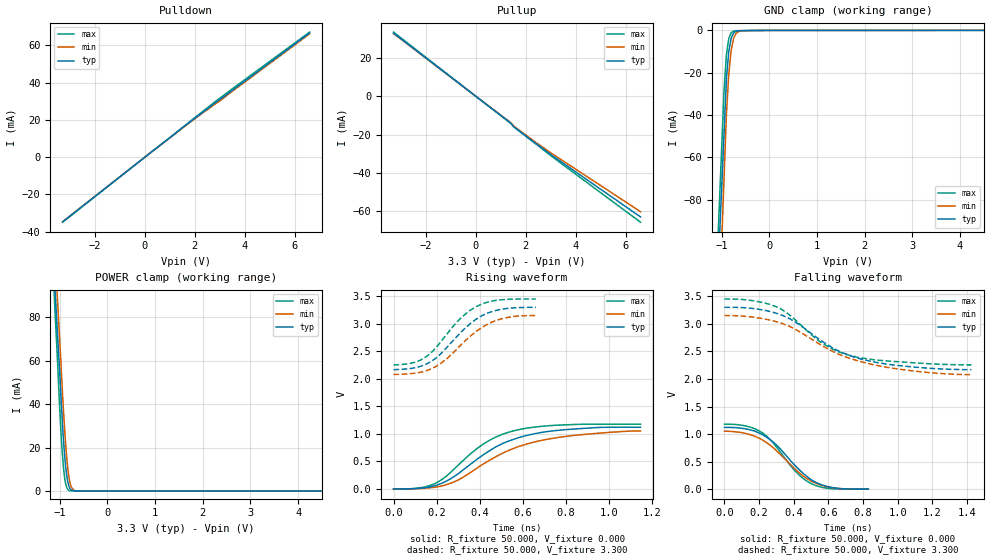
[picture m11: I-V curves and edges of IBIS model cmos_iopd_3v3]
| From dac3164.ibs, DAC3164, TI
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[Model]   cmos_iopd_3v3
Model_type I/O
Vinl=8.250E-01
Vinh=1.980E+00
Vref=0.000E+00
Rref=1.000E+06
Cref=0.000E+00
Vmeas=1.650E+00
C_comp   1.070E-12   1.070E-12   1.070E-12
[Voltage Range]   3.300E+00   3.150E+00   3.450E+00
[POWER Clamp Reference]   3.300E+00   3.150E+00   3.450E+00
[GND Clamp Reference]   0.000E+00   0.000E+00   0.000E+00
[Pullup Reference]   3.300E+00   3.150E+00   3.450E+00
[Pulldown Reference]   0.000E+00   0.000E+00   0.000E+00
[Temperature Range]   25   85   -40
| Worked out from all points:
|   slope of the pulldown table from 0 to 0.495 V, typ, clamps not added: 95.4 ohm
|   slope of the pullup table from 0 to 0.495 V, typ, clamps not added: 100 ohm
|   GND clamp passes 1 mA (typ) near -0.74 V on its own axis
|   POWER clamp passes 1 mA (typ) near -0.78 V on its own axis
|   rising waveform, R_fixture 50.000, V_fixture 0.000: 20-80 % time 273ps typ, 321ps min, 229ps max; typ from 0 V to 1.12 V
|   falling waveform, R_fixture 50.000, V_fixture 0.000: 20-80 % time 214ps typ, 223ps min, 189ps max; typ from 1.12 V to 0 V
|   rising waveform, R_fixture 50.000, V_fixture 3.300: 20-80 % time 178ps typ, 188ps min, 165ps max; typ from 2.17 V to 3.3 V
|   falling waveform, R_fixture 50.000, V_fixture 3.300: 20-80 % time 365ps typ, 424ps min, 305ps max; typ from 3.3 V to 2.17 V
[GND Clamp]
-3.3V     -1.265A    -1.499A    -1.32A
-950mV    -49.06mA   -70.33mA   -28.61mA
-900mV    -23.2mA    -39.94mA   -11.61mA
-850mV    -9.95mA    -20.84mA   -3.839mA
-800mV    -3.735mA   -9.456mA   -1.133mA
-750mV    -1.255mA   -3.879mA   -337.2uA
-700mV    -399.4uA   -1.494mA   -148.9uA
-650mV    -154.5uA   -584.3uA   -131.2uA
-600mV    -133.2uA   -198.5uA   -113.5uA
-300mV    -15.44uA   -31.58uA   -24.54uA
6.6V      32.89uA    44.03uA    40.1uA
[Power Clamp]
-3.3V     957.2mA    1.007A     1.073A
-1.1V     92.68mA    109.2mA    82.9mA
-1.06V    76.96mA    92.93mA    65.21mA
-1.04V    69.1mA     84.79mA    56.18mA
-980mV    45.39mA    60.51mA    28.92mA
-940mV    29.43mA    43.6mA     15.23mA
-880mV    11.72mA    22.38mA    3.527mA
-840mV    5.021mA    12.01mA    880.7uA
-800mV    1.611mA    5.206mA    167.9uA
-760mV    445uA      1.789mA    28uA
-640mV    29.31uA    9.511uA    16.77uA
6.6V      0A         0A         0A
[Pullup]
-3.3V     33mA       32.76mA    33.52mA
1.36V     -13.56mA   -13.33mA   -13.75mA
1.52V     -15.88mA   -15.57mA   -15.97mA
2.42V     -24.71mA   -24.19mA   -25mA
3.08V     -31.11mA   -30.16mA   -31.67mA
6.6V      -62.94mA   -60.21mA   -65.7mA
[Pulldown]
-3.3V     -34.84mA   -34.69mA   -34.99mA
1.48V     15.55mA    15.35mA    15.69mA
2.82V     29.19mA    28.62mA    29.86mA
6.6V      66.72mA    66.24mA    67.21mA
[Rising Waveform]
R_fixture = 50.000
V_fixture = 0.000
V_fixture_min = 0.000
V_fixture_max = 0.000
|  time   V(typ)   V(min)   V(max)
0s        435.7uV    927.3uV    -4.246mV
120ps     11.99mV    6.341mV    19.28mV
195ps     62.56mV    32.43mV    104.3mV
300ps     277.3mV    163.1mV    433mV
410ps     604.1mV    437.5mV    798.5mV
475ps     764.1mV    587.5mV    943.7mV
550ps     892.5mV    726.3mV    1.049V
665ps     1.012V     863.7mV    1.129V
790ps     1.074V     950.1mV    1.164V
1.145ns   1.121V     1.053V     1.176V
[Falling Waveform]
R_fixture = 50.000
V_fixture = 0.000
V_fixture_min = 0.000
V_fixture_max = 0.000
|  time   V(typ)   V(min)   V(max)
0s        1.121V     1.053V     1.179V
125ps     1.092V     1.009V     1.145V
220ps     987.8mV    891.2mV    1.02V
300ps     801.4mV    699.1mV    765.1mV
420ps     388.6mV    328mV      291.6mV
465ps     259.3mV    216mV      169.1mV
510ps     154mV      133.5mV    88.15mV
565ps     75.22mV    64.94mV    32.04mV
635ps     22.94mV    19.9mV     4.413mV
830ps     435.7uV    927.3uV    708.3uV
[Rising Waveform]
R_fixture = 50.000
V_fixture = 3.300
V_fixture_min = 3.150
V_fixture_max = 3.450
|  time   V(typ)   V(min)   V(max)
0s        2.168V     2.08V      2.255V
105ps     2.207V     2.107V     2.31V
175ps     2.318V     2.183V     2.479V
245ps     2.562V     2.359V     2.802V
305ps     2.816V     2.587V     3.077V
350ps     2.984V     2.755V     3.23V
395ps     3.114V     2.894V     3.334V
450ps     3.214V     3.02V      3.408V
515ps     3.273V     3.105V     3.442V
660ps     3.3V       3.15V      3.45V
[Falling Waveform]
R_fixture = 50.000
V_fixture = 3.300
V_fixture_min = 3.150
V_fixture_max = 3.450
|  time   V(typ)   V(min)   V(max)
0s        3.3V       3.15V      3.45V
160ps     3.28V      3.124V     3.422V
300ps     3.192V     3.039V     3.309V
405ps     3.041V     2.908V     3.083V
565ps     2.681V     2.602V     2.648V
640ps     2.537V     2.477V     2.519V
725ps     2.424V     2.372V     2.427V
990ps     2.248V     2.186V     2.315V
1.205ns   2.19V      2.109V     2.272V
1.425ns   2.168V     2.08V      2.255V
[Ramp]
dV/dt_r   6.7298E-01/2.7256E-10   6.2996E-01/3.2059E-10   7.0820E-01/2.2857E-10
dV/dt_f   6.7918E-01/3.6465E-10   6.4206E-01/4.2404E-10   7.1696E-01/3.0414E-10
R_load = 50
